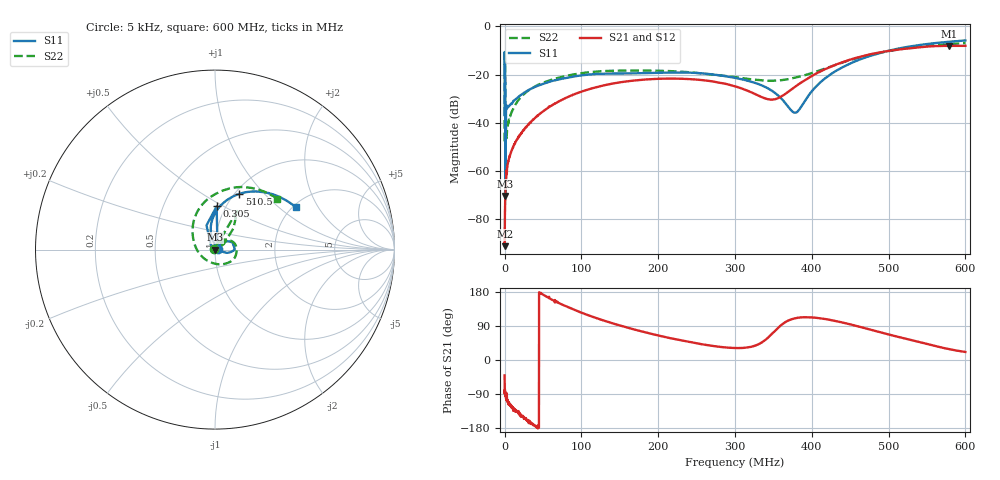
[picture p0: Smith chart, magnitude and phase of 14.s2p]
#  HZ  S  MA  R  50.00
! Rohde & Schwarz Vector Network Analyzer
! Rohde-Schwarz,ZNL6-2Port,1323001206101378,1.50.1.34-21.10.1.104
! Created: UTC 1/22/2024, 9:08:22 AM
! freq[Hz]  mag:S11  ang:S11  mag:S21  ang:S21  mag:S12  ang:S12  mag:S22  ang:S22
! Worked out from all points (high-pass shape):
!   6000 points, 5 kHz to 600 MHz, reference 50 ohm
!   highest |S21| = -8.11 dB at 578.8 MHz (marker M1); lowest = -91.1 dB at 105 kHz (marker M2)
!   |S21| within 3 dB of the highest: 483.5 MHz to end of sweep
!   lowest |S11| = -70.3 dB at 1.105 MHz (marker M3), VSWR 1.00, Z = 50 + j0.0211 ohm
!   |S11| at or under -10 dB: start of sweep to 501.8 MHz
!   |S22| runs from -47.7 to -7.0 dB; largest |S21 - S12| = 0.015
!   S11 on the Smith chart (normalised r, x): 5 kHz: 1.03, +0.01; 305 kHz: 0.91, +0.46; 510.5 MHz: 1.05, +0.74; 600 MHz: 2.07, +1.32
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5000  0.01486 16.4  3.229e-05 -40.7  4.495e-05 -71.6  0.004143 145.0
105015.8  0.293 72.0  2.798e-05 -83.3  4.571e-05 -60.7  0.2864 74.0
305047.5  0.241 87.8  9.521e-05 -87.0  0.0001008 -95.6  0.2476 60.1
1105174  0.0003072 136.7  0.0004224 -95.2  0.0003921 -90.1  0.02504 19.4
3105491  0.01991 15.6  0.001108 -106.2  0.00112 -106.9  0.006857 70.8
3905618  0.02068 18.1  0.001367 -105.8  0.001316 -114.4  0.00816 71.0
6305998  0.02278 24.6  0.00198 -117.3  0.001976 -117.6  0.01217 70.5
1.2607e7  0.02931 34.7  0.003542 -132.5  0.003576 -128.2  0.02179 69.5
2.250856e7  0.03899 42.2  0.006301 -148.8  0.006466 -146.9  0.0357 66.1
5.581384e7  0.06864 40.1  0.02006 165.9  0.01992 163.9  0.07328 49.1
1.000208e8  0.09609 27.3  0.04428 124.9  0.04397 122.9  0.1067 25.0
2.000367e8  0.1083 6.2  0.08158 64.8  0.08118 63.1  0.1197 -18.5
2.555455e8  0.1062 -1.9  0.07717 42.0  0.07694 40.4  0.1062 -41.5
3.000525e8  0.0854 -10.2  0.05709 31.6  0.0568 30.0  0.08845 -68.1
3.4736e8  0.04691 -15.8  0.03021 67.4  0.03002 65.4  0.07436 -117.2
3.774648e8  0.01625 37.8  0.05474 109.7  0.05453 107.6  0.08529 -157.8
4.000683e8  0.0451 102.3  0.09359 112.4  0.09315 110.3  0.1075 173.7
4.389745e8  0.1388 99.3  0.178 99.4  0.1774 97.6  0.1764 134.8
5.000842e8  0.3116 71.4  0.3084 67.4  0.3057 66.1  0.3059 90.9
5.104858e8  0.3395 66.3  0.3252 62.0  0.3237 61.0  0.3263 84.2
5.787966e8  0.4777 35.8  0.3929 28.6  0.3878 27.5  0.427 48.3
6e8  0.5078 27.6  0.3927 21.2  0.3936 20.7  0.4481 39.1
